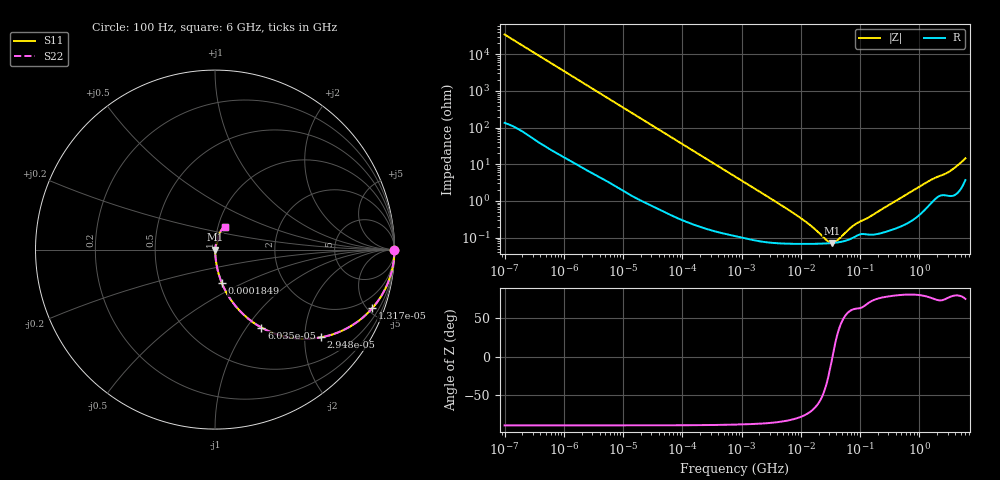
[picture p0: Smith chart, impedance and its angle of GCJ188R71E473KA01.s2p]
!Murata Part Number: GCJ188R71E473KA01
!These Parameters are Measured in Series Mode Connection
!Data Generated on Mar 13, 2026
!  o--ll--o
!Port1  Port2
!  o------o
!Operation Temp=25[degC], DC Bias Voltage=0[V]
!Freq. Start=100[Hz] Stop=6[GHz] 401[Steps]
# Hz S RI R 50
!Freq.(Hz) S11(Real) S11(Imag) S21(Real) S21(Imag) S12(Real) S12(Imag) S22(Real) S22(Imag)
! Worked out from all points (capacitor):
!   401 points, 100 Hz to 6 GHz, reference 50 ohm
!   read as one part in series: C = 45.7 nF near 109 Hz
!   lowest |Z| = 71.2 mohm at 33.3 MHz (marker M1)
!   series resonance near 34.22 MHz, so ESL is about 470 pH
!   S11 on the Smith chart (normalised r, x): 100 Hz: open; 13.17 kHz: 1.03, -5.36; 29.48 kHz: 1.02, -2.40; 60.35 kHz: 1.01, -1.18; 184.9 kHz: 1.00, -0.39; 6 GHz: 1.07, +0.28
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100  1 -0.00288  1.94e-05 0.00288  1.94e-05 0.00288  1 -0.00288
2008  0.9965 -0.057  0.00353 0.057  0.00353 0.057  0.9965 -0.057
5378  0.9764 -0.1491  0.0236 0.1491  0.0236 0.1491  0.9764 -0.1491
13169  0.8765 -0.3263  0.1235 0.3263  0.1235 0.3263  0.8765 -0.3263
19704  0.7616 -0.4232  0.2384 0.4232  0.2384 0.4232  0.7616 -0.4232
29482  0.5898 -0.4887  0.4102 0.4887  0.4102 0.4887  0.5898 -0.4887
40335  0.436 -0.4925  0.564 0.4925  0.564 0.4925  0.436 -0.4925
60352  0.2585 -0.4342  0.7415 0.4342  0.7415 0.4342  0.2585 -0.4342
98762  0.1168 -0.317  0.8832 0.317  0.8832 0.317  0.1168 -0.317
184852  0.0377 -0.1852  0.9623 0.1852  0.9623 0.1852  0.0377 -0.1852
361830  0.0111 -0.0976  0.9889 0.0976  0.9889 0.0976  0.0111 -0.0976
774597  0.00324 -0.0462  0.9968 0.0462  0.9968 0.0462  0.00324 -0.0462
6075234  0.000714 -0.00578  0.9993 0.00578  0.9993 0.00578  0.000714 -0.00578
1.555665e7  0.000677 -0.00185  0.9993 0.00185  0.9993 0.00185  0.000677 -0.00185
2.784235e7  0.000694 -0.00044  0.9993 0.00044  0.9993 0.00044  0.000694 -0.00044
3.330331e7  0.000709 -5.73e-05  0.9993 5.73e-05  0.9993 5.73e-05  0.000709 -5.73e-05
3.983537e7  0.000731 0.000324  0.9993 -0.000324  0.9993 -0.000324  0.000731 0.000324
8.527865e7  0.0011 0.0021  0.9989 -0.0021  0.9989 -0.0021  0.0011 0.0021
3.124326e8  0.0016 0.00773  0.9984 -0.00773  0.9984 -0.00773  0.0016 0.00773
1.431855e9  0.00836 0.0332  0.9916 -0.0332  0.9916 -0.0332  0.00836 0.0332
3.065283e9  0.017 0.0571  0.983 -0.0571  0.983 -0.0571  0.017 0.0571
6e9  0.0532 0.1286  0.9468 -0.1286  0.9468 -0.1286  0.0532 0.1286
